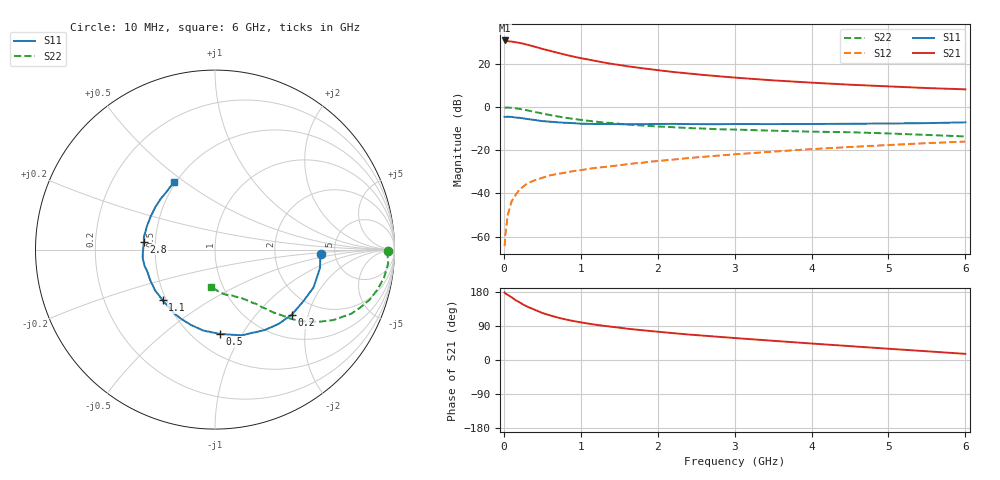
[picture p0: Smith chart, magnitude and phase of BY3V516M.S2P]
! SIEMENS Small Signal Semiconductors
! BFY420
! Si NPN RF SIEGET Grounded Emitter Transistor in MICRO-X
! VCE = 3.5 V  IC = 16 mA
! Common Emitter S-Parameters:  October  1996
# GHz  S  MA  R  50
!  f  S11  S21  S12  S22
! GHz  MAG  ANG  MAG  ANG  MAG  ANG  MAG  ANG
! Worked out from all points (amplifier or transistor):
!   36 points, 10 MHz to 6 GHz, reference 50 ohm
!   highest |S21| = 30.8 dB at 10 MHz (marker M1)
!   |S21| within 3 dB of that: start of sweep to 413.1 MHz
!   unconditionally stable (mu >= 1): start of sweep to 16.14 MHz; 2.169 GHz to end of sweep
!   at 250 MHz: K = 0.28, MSG = 33.1 dB, |S12| = -36.9 dB
!   at 1.4 GHz: K = 0.86, MSG = 23.7 dB, |S12| = -27.4 dB
!   at 6 GHz: K = 1.07, MAG = 10.5 dB, |S12| = -16.0 dB
!   S11 on the Smith chart (normalised r, x): 10 MHz: 3.86, -0.27; 200 MHz: 1.49, -1.58; 500 MHz: 0.67, -0.80; 1.1 GHz: 0.48, -0.32; 2.8 GHz: 0.43, +0.05; 6 GHz: 0.49, +0.45
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0.01  0.5898 -2.2  34.57 178.4  0.0006 60.8  0.9664 -0.5
0.02  0.5884 -4.1  34.15 175.8  0.0011 66.4  0.9615 -1.5
0.05  0.5938 -10.0  33.18 171.9  0.0031 84.3  0.9679 -4.5
0.1  0.5881 -21.1  32.63 165.7  0.0065 77.1  0.9545 -9.5
0.15  0.5698 -30.5  31.51 158.3  0.009 73.3  0.9311 -14.0
0.2  0.5607 -40.4  30.46 152.8  0.0121 72.5  0.9053 -18.0
0.25  0.5447 -49.6  29.14 146.5  0.0143 68.5  0.871 -21.8
0.3  0.527 -58.2  27.71 141.3  0.0167 67.3  0.8391 -25.2
0.4  0.5003 -72.8  24.86 132.6  0.0201 62.6  0.7683 -30.7
0.5  0.4706 -86.7  22.08 124.1  0.0229 60.4  0.7049 -34.8
0.6  0.4558 -98.2  19.9 117.8  0.0261 58.1  0.6498 -38.1
0.7  0.4405 -107.7  17.93 112.1  0.0282 57.8  0.6037 -40.8
0.8  0.4297 -115.9  16.16 107.2  0.0302 56.0  0.5627 -42.8
0.9  0.4225 -122.6  14.7 103.0  0.0327 55.5  0.5302 -44.1
1.1  0.4065 -135.9  12.49 96.0  0.0369 56.3  0.4781 -47.1
1.6  0.3977 -157.4  8.777 82.7  0.0471 56.1  0.3929 -52.0
2.2  0.4056 -173.9  6.453 70.9  0.0605 55.1  0.34 -57.1
2.8  0.3988 173.6  5.12 61.1  0.0751 53.0  0.3042 -61.8
3.5  0.4011 160.8  4.122 50.7  0.0926 49.3  0.2818 -67.3
4.5  0.4077 145.3  3.271 36.6  0.1183 42.2  0.2598 -75.9
5.5  0.4221 128.6  2.736 23.0  0.1453 33.8  0.2251 -88.3
6  0.4403 121.5  2.557 16.2  0.1581 29.2  0.2076 -96.4
